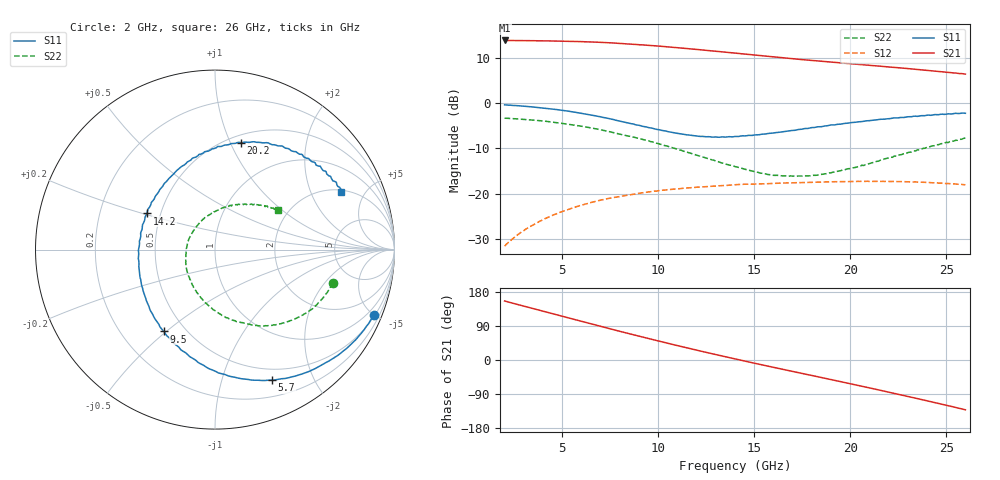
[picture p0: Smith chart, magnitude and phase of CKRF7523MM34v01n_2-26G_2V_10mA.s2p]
! CHUO DENSHI KOGYO Co.,Ltd.
! 8. March 2017
! CKRF7523MM34_RT5880
! N-channel HJ-FET
! Vds = 2 V Id = 10 mA
# Hz S  MA  R 50
!	f	S11	S21	S12	S22
!	Hz	MAG	ANG	MAG	ANG	MAG	ANG	MAG	ANG
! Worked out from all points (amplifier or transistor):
!   241 points, 2 GHz to 26 GHz, reference 50 ohm
!   highest |S21| = 13.9 dB at 2 GHz (marker M1)
!   |S21| within 3 dB of that: start of sweep to 14.49 GHz
!   unconditionally stable (mu >= 1): 12.92 GHz to 18.93 GHz
!   at 6 GHz: K = 0.60, MSG = 18.1 dB, |S12| = -22.5 dB
!   at 14 GHz: K = 1.02, MAG = 13.8 dB, |S12| = -18.0 dB
!   at 26 GHz: K = 0.77, MSG = 12.2 dB, |S12| = -18.0 dB
!   lowest NFmin = 0.34 dB at 10 GHz
!   S11 on the Smith chart (normalised r, x): 2 GHz: 0.56, -5.02; 5.7 GHz: 0.37, -1.46; 9.5 GHz: 0.38, -0.49; 14.2 GHz: 0.42, +0.21; 20.2 GHz: 0.57, +1.09; 26 GHz: 2.10, +3.36
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2e9  0.9585 -22.2  4.931 155.8  0.02633 77.0  0.6825 -15.8
2.8e9  0.9342 -31.5  4.916 144.8  0.03679 70.4  0.6667 -21.6
3.8e9  0.8923 -43.1  4.894 131.5  0.04934 62.8  0.6415 -29.2
4.8e9  0.8453 -55.1  4.861 118.2  0.06129 55.2  0.6055 -37.4
5.7e9  0.7923 -66.5  4.808 106.2  0.07141 48.4  0.5686 -45.0
6e9  0.7733 -70.5  4.786 102.2  0.07471 46.1  0.5555 -47.5
6.7e9  0.7271 -79.8  4.729 92.9  0.08192 40.9  0.5231 -53.8
7.5e9  0.6707 -91.3  4.649 82.3  0.08945 34.9  0.4821 -61.2
8.5e9  0.5978 -105.8  4.498 69.3  0.09701 28.3  0.4319 -70.3
9.5e9  0.5372 -121.9  4.356 56.6  0.1046 21.5  0.3837 -80.8
1e10  0.5109 -130.8  4.271 50.3  0.1078 18.1  0.3579 -86.1
1.1e10  0.4642 -148.7  4.101 38.0  0.1132 11.8  0.3096 -97.8
1.2e10  0.4346 -167.5  3.927 26.0  0.1181 5.8  0.2667 -110.5
1.3e10  0.424 173.6  3.746 14.3  0.1216 0.1  0.2291 -124.3
1.4e10  0.4291 155.4  3.574 2.9  0.1256 -5.5  0.1992 -140.3
1.42e10  0.4292 152.0  3.542 0.6  0.1267 -6.8  0.1946 -144.1
1.63e10  0.4772 120.0  3.205 -22.6  0.1305 -18.5  0.1583 176.1
1.8e10  0.5378 99.5  2.968 -40.9  0.1336 -27.6  0.1578 141.3
2.02e10  0.6134 76.6  2.711 -64.8  0.1365 -40.4  0.194 101.4
2.2e10  0.6738 59.6  2.514 -84.8  0.1366 -52.1  0.2487 75.1
2.39e10  0.7284 42.3  2.316 -106.5  0.1335 -64.9  0.318 52.3
2.6e10  0.7735 24.5  2.095 -131.4  0.1256 -80.7  0.4127 32.3
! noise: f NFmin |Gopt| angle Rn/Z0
1e+10  0.34  0.438  91.2  0.09
1.05e+10  0.36  0.423  97  0.08
1.1e+10  0.38  0.405  106  0.07
1.15e+10  0.4  0.385  113.8  0.06
1.2e+10  0.42  0.364  123.3  0.06
1.25e+10  0.44  0.351  134.9  0.05
1.3e+10  0.46  0.341  144.6  0.04
1.35e+10  0.48  0.33  157.4  0.04
1.4e+10  0.5  0.329  170.3  0.04
1.5e+10  0.54  0.332  -165.7  0.04
